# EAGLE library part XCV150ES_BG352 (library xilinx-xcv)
xcv150es_bg352 edit this description Auto generated by make-symbol-device-package-bsdl.ulp Rev. 26 Source: xcv150es_bg352.bsd
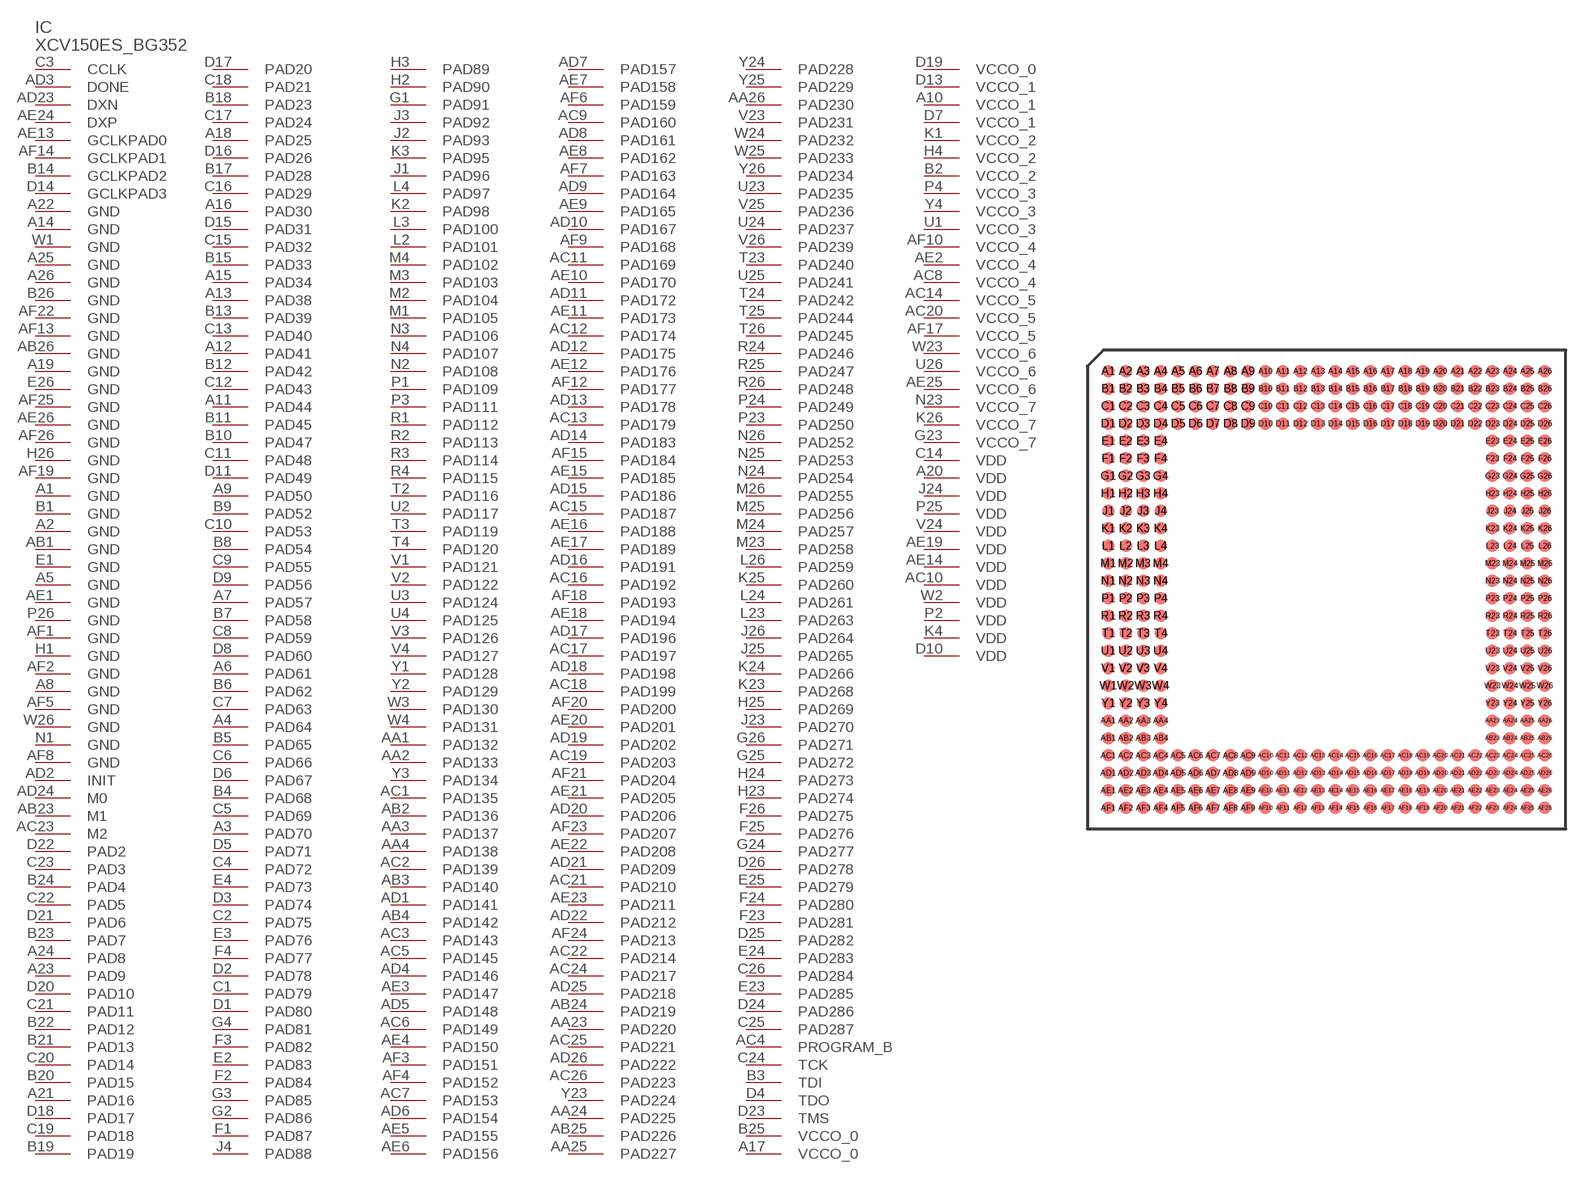
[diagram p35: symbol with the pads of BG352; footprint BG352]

Designator prefix IC

## XCV150ES_BG352 (OC_FARNELL: unknown; OC_NEWARK: unknown)  [BG352]
A1  GND  pwr
A2  GND  pwr
A3  PAD70
A4  PAD64
A5  GND  pwr
A6  PAD61
A7  PAD57
A8  GND  pwr
A9  PAD50
A10  VCCO_1  pwr
A11  PAD44
A12  PAD41
A13  PAD38
A14  GND  pwr
A15  PAD34
A16  PAD30
A17  VCCO_0  pwr
A18  PAD25
A19  GND  pwr
A20  VDD  pwr
A21  PAD16
A22  GND  pwr
A23  PAD9
A24  PAD8
A25  GND  pwr
A26  GND  pwr
AA1  PAD132
AA2  PAD133
AA3  PAD137
AA4  PAD138
AA23  PAD220
AA24  PAD225
AA25  PAD227
AA26  PAD230
AB1  GND  pwr
AB2  PAD136
AB3  PAD140
AB4  PAD142
AB23  M1  in
AB24  PAD219
AB25  PAD226
AB26  GND  pwr
AC1  PAD135
AC2  PAD139
AC3  PAD143
AC4  PROGRAM_B  in
AC5  PAD145
AC6  PAD149
AC7  PAD153
AC8  VCCO_4  pwr
AC9  PAD160
AC10  VDD  pwr
AC11  PAD169
AC12  PAD174
AC13  PAD179
AC14  VCCO_5  pwr
AC15  PAD187
AC16  PAD192
AC17  PAD197
AC18  PAD199
AC19  PAD203
AC20  VCCO_5  pwr
AC21  PAD210
AC22  PAD214
AC23  M2  in
AC24  PAD217
AC25  PAD221
AC26  PAD223
AD1  PAD141
AD2  INIT
AD3  DONE
AD4  PAD146
AD5  PAD148
AD6  PAD154
AD7  PAD157
AD8  PAD161
AD9  PAD164
AD10  PAD167
AD11  PAD172
AD12  PAD175
AD13  PAD178
AD14  PAD183
AD15  PAD186
AD16  PAD191
AD17  PAD196
AD18  PAD198
AD19  PAD202
AD20  PAD206
AD21  PAD209
AD22  PAD212
AD23  DXN  pas
AD24  M0  in
AD25  PAD218
AD26  PAD222
AE1  GND  pwr
AE2  VCCO_4  pwr
AE3  PAD147
AE4  PAD150
AE5  PAD155
AE6  PAD156
AE7  PAD158
AE8  PAD162
AE9  PAD165
AE10  PAD170
AE11  PAD173
AE12  PAD176
AE13  GCLKPAD0  in
AE14  VDD  pwr
AE15  PAD185
AE16  PAD188
AE17  PAD189
AE18  PAD194
AE19  VDD  pwr
AE20  PAD201
AE21  PAD205
AE22  PAD208
AE23  PAD211
AE24  DXP  pas
AE25  VCCO_6  pwr
AE26  GND  pwr
AF1  GND  pwr
AF2  GND  pwr
AF3  PAD151
AF4  PAD152
AF5  GND  pwr
AF6  PAD159
AF7  PAD163
AF8  GND  pwr
AF9  PAD168
AF10  VCCO_4  pwr
AF12  PAD177
AF13  GND  pwr
AF14  GCLKPAD1  in
AF15  PAD184
AF17  VCCO_5  pwr
AF18  PAD193
AF19  GND  pwr
AF20  PAD200
AF21  PAD204
AF22  GND  pwr
AF23  PAD207
AF24  PAD213
AF25  GND  pwr
AF26  GND  pwr
B1  GND  pwr
B2  VCCO_2  pwr
B3  TDI  in
B4  PAD68
B5  PAD65
B6  PAD62
B7  PAD58
B8  PAD54
B9  PAD52
B10  PAD47
B11  PAD45
B12  PAD42
B13  PAD39
B14  GCLKPAD2  in
B15  PAD33
B17  PAD28
B18  PAD23
B19  PAD19
B20  PAD15
B21  PAD13
B22  PAD12
B23  PAD7
B24  PAD4
B25  VCCO_0  pwr
B26  GND  pwr
C1  PAD79
C2  PAD75
C3  CCLK
C4  PAD72
C5  PAD69
C6  PAD66
C7  PAD63
C8  PAD59
C9  PAD55
C10  PAD53
C11  PAD48
C12  PAD43
C13  PAD40
C14  VDD  pwr
C15  PAD32
C16  PAD29
C17  PAD24
C18  PAD21
C19  PAD18
C20  PAD14
C21  PAD11
C22  PAD5
C23  PAD3
C24  TCK  in
C25  PAD287
C26  PAD284
D1  PAD80
D2  PAD78
D3  PAD74
D4  TDO  out
D5  PAD71
D6  PAD67
D7  VCCO_1  pwr
D8  PAD60
D9  PAD56
D10  VDD  pwr
D11  PAD49
D13  VCCO_1  pwr
D14  GCLKPAD3  in
D15  PAD31
D16  PAD26
D17  PAD20
D18  PAD17
D19  VCCO_0  pwr
D20  PAD10
D21  PAD6
D22  PAD2
D23  TMS  in
D24  PAD286
D25  PAD282
D26  PAD278
E1  GND  pwr
E2  PAD83
E3  PAD76
E4  PAD73
E23  PAD285
E24  PAD283
E25  PAD279
E26  GND  pwr
F1  PAD87
F2  PAD84
F3  PAD82
F4  PAD77
F23  PAD281
F24  PAD280
F25  PAD276
F26  PAD275
G1  PAD91
G2  PAD86
G3  PAD85
G4  PAD81
G23  VCCO_7  pwr
G24  PAD277
G25  PAD272
G26  PAD271
H1  GND  pwr
H2  PAD90
H3  PAD89
H4  VCCO_2  pwr
H23  PAD274
H24  PAD273
H25  PAD269
H26  GND  pwr
J1  PAD96
J2  PAD93
J3  PAD92
J4  PAD88
J23  PAD270
J24  VDD  pwr
J25  PAD265
J26  PAD264
K1  VCCO_2  pwr
K2  PAD98
K3  PAD95
K4  VDD  pwr
K23  PAD268
K24  PAD266
K25  PAD260
K26  VCCO_7  pwr
L2  PAD101
L3  PAD100
L4  PAD97
L23  PAD263
L24  PAD261
L26  PAD259
M1  PAD105
M2  PAD104
M3  PAD103
M4  PAD102
M23  PAD258
M24  PAD257
M25  PAD256
M26  PAD255
N1  GND  pwr
N2  PAD108
N3  PAD106
N4  PAD107
N23  VCCO_7  pwr
N24  PAD254
N25  PAD253
N26  PAD252
P1  PAD109
P2  VDD  pwr
P3  PAD111
P4  VCCO_3  pwr
P23  PAD250
P24  PAD249
P25  VDD  pwr
P26  GND  pwr
R1  PAD112
R2  PAD113
R3  PAD114
R4  PAD115
R24  PAD246
R25  PAD247
R26  PAD248
T2  PAD116
T3  PAD119
T4  PAD120
T23  PAD240
T24  PAD242
T25  PAD244
T26  PAD245
U1  VCCO_3  pwr
U2  PAD117
U3  PAD124
U4  PAD125
U23  PAD235
U24  PAD237
U25  PAD241
U26  VCCO_6  pwr
V1  PAD121
V2  PAD122
V3  PAD126
V4  PAD127
V23  PAD231
V24  VDD  pwr
V25  PAD236
V26  PAD239
W1  GND  pwr
W2  VDD  pwr
W3  PAD130
W4  PAD131
W23  VCCO_6  pwr
W24  PAD232
W25  PAD233
W26  GND  pwr
Y1  PAD128
Y2  PAD129
Y3  PAD134
Y4  VCCO_3  pwr
Y23  PAD224
Y24  PAD228
Y25  PAD229
Y26  PAD234

## Footprint BG352 (pad centres in mm)
xcv100e_bg352 edit this description Auto generated by make-symbol-device-package-bsdl.ulp Rev. 26 Source: xcv100e_bg352.bsd
smd 0.9 x 0.9: A1 -15.875,15.875; A2 -14.605,15.875; A3 -13.335,15.875; A4 -12.065,15.875; A5 -10.795,15.875; A6 -9.525,15.875; A7 -8.255,15.875; A8 -6.985,15.875; A9 -5.715,15.875; A10 -4.445,15.875; A11 -3.175,15.875; A12 -1.905,15.875; A13 -0.635,15.875; A14 0.635,15.875; A15 1.905,15.875; A16 3.175,15.875; A17 4.445,15.875; A18 5.715,15.875; A19 6.985,15.875; A20 8.255,15.875; A21 9.525,15.875; A22 10.795,15.875; A23 12.065,15.875; A24 13.335,15.875; A25 14.605,15.875; A26 15.875,15.875; AA1 -15.875,-9.525; AA2 -14.605,-9.525; AA3 -13.335,-9.525; AA4 -12.065,-9.525; AA23 12.065,-9.525; AA24 13.335,-9.525; AA25 14.605,-9.525; AA26 15.875,-9.525; AB1 -15.875,-10.795; AB2 -14.605,-10.795; AB3 -13.335,-10.795; AB4 -12.065,-10.795; AB23 12.065,-10.795; AB24 13.335,-10.795; AB25 14.605,-10.795; AB26 15.875,-10.795; AC1 -15.875,-12.065; AC2 -14.605,-12.065; AC3 -13.335,-12.065; AC4 -12.065,-12.065; AC5 -10.795,-12.065; AC6 -9.525,-12.065; AC7 -8.255,-12.065; AC8 -6.985,-12.065; AC9 -5.715,-12.065; AC10 -4.445,-12.065; AC11 -3.175,-12.065; AC12 -1.905,-12.065; AC13 -0.635,-12.065; AC14 0.635,-12.065; AC15 1.905,-12.065; AC16 3.175,-12.065; AC17 4.445,-12.065; AC18 5.715,-12.065; AC19 6.985,-12.065; AC20 8.255,-12.065; AC21 9.525,-12.065; AC22 10.795,-12.065; AC23 12.065,-12.065; AC24 13.335,-12.065; AC25 14.605,-12.065; AC26 15.875,-12.065; AD1 -15.875,-13.335; AD2 -14.605,-13.335; AD3 -13.335,-13.335; AD4 -12.065,-13.335; AD5 -10.795,-13.335; AD6 -9.525,-13.335; AD7 -8.255,-13.335; AD8 -6.985,-13.335; AD9 -5.715,-13.335; AD10 -4.445,-13.335; AD11 -3.175,-13.335; AD12 -1.905,-13.335; AD13 -0.635,-13.335; AD14 0.635,-13.335; AD15 1.905,-13.335; AD16 3.175,-13.335; AD17 4.445,-13.335; AD18 5.715,-13.335; AD19 6.985,-13.335; AD20 8.255,-13.335; AD21 9.525,-13.335; AD22 10.795,-13.335; AD23 12.065,-13.335; AD24 13.335,-13.335; AD25 14.605,-13.335; AD26 15.875,-13.335; AE1 -15.875,-14.605; AE2 -14.605,-14.605; AE3 -13.335,-14.605; AE4 -12.065,-14.605; AE5 -10.795,-14.605; AE6 -9.525,-14.605; AE7 -8.255,-14.605; AE8 -6.985,-14.605; AE9 -5.715,-14.605; AE10 -4.445,-14.605; AE11 -3.175,-14.605; AE12 -1.905,-14.605; AE13 -0.635,-14.605; AE14 0.635,-14.605; AE15 1.905,-14.605; AE16 3.175,-14.605; AE17 4.445,-14.605; AE18 5.715,-14.605; AE19 6.985,-14.605; AE20 8.255,-14.605; AE21 9.525,-14.605; AE22 10.795,-14.605; AE23 12.065,-14.605; AE24 13.335,-14.605; AE25 14.605,-14.605; AE26 15.875,-14.605; AF1 -15.875,-15.875; AF2 -14.605,-15.875; AF3 -13.335,-15.875; AF4 -12.065,-15.875; AF5 -10.795,-15.875; AF6 -9.525,-15.875; AF7 -8.255,-15.875; AF8 -6.985,-15.875; AF9 -5.715,-15.875; AF10 -4.445,-15.875; AF11 -3.175,-15.875; AF12 -1.905,-15.875; AF13 -0.635,-15.875; AF14 0.635,-15.875; AF15 1.905,-15.875; AF16 3.175,-15.875; AF17 4.445,-15.875; AF18 5.715,-15.875; AF19 6.985,-15.875; AF20 8.255,-15.875; AF21 9.525,-15.875; AF22 10.795,-15.875; AF23 12.065,-15.875; AF24 13.335,-15.875; AF25 14.605,-15.875; AF26 15.875,-15.875; B1 -15.875,14.605; B2 -14.605,14.605; B3 -13.335,14.605; B4 -12.065,14.605; B5 -10.795,14.605; B6 -9.525,14.605; B7 -8.255,14.605; B8 -6.985,14.605; B9 -5.715,14.605; B10 -4.445,14.605; B11 -3.175,14.605; B12 -1.905,14.605; B13 -0.635,14.605; B14 0.635,14.605; B15 1.905,14.605; B16 3.175,14.605; B17 4.445,14.605; B18 5.715,14.605; B19 6.985,14.605; B20 8.255,14.605; B21 9.525,14.605; B22 10.795,14.605; B23 12.065,14.605; B24 13.335,14.605; B25 14.605,14.605; B26 15.875,14.605; C1 -15.875,13.335; C2 -14.605,13.335; C3 -13.335,13.335; C4 -12.065,13.335; C5 -10.795,13.335; C6 -9.525,13.335; C7 -8.255,13.335; C8 -6.985,13.335; C9 -5.715,13.335; C10 -4.445,13.335; C11 -3.175,13.335; C12 -1.905,13.335; C13 -0.635,13.335; C14 0.635,13.335; C15 1.905,13.335; C16 3.175,13.335; C17 4.445,13.335; C18 5.715,13.335; C19 6.985,13.335; C20 8.255,13.335; C21 9.525,13.335; C22 10.795,13.335; C23 12.065,13.335; C24 13.335,13.335; C25 14.605,13.335; C26 15.875,13.335; D1 -15.875,12.065; D2 -14.605,12.065; D3 -13.335,12.065; D4 -12.065,12.065; D5 -10.795,12.065; D6 -9.525,12.065; D7 -8.255,12.065; D8 -6.985,12.065; D9 -5.715,12.065; D10 -4.445,12.065; D11 -3.175,12.065; D12 -1.905,12.065; D13 -0.635,12.065; D14 0.635,12.065; D15 1.905,12.065; D16 3.175,12.065; D17 4.445,12.065; D18 5.715,12.065; D19 6.985,12.065; D20 8.255,12.065; D21 9.525,12.065; D22 10.795,12.065; D23 12.065,12.065; D24 13.335,12.065; D25 14.605,12.065; D26 15.875,12.065; E1 -15.875,10.795; E2 -14.605,10.795; E3 -13.335,10.795; E4 -12.065,10.795; E23 12.065,10.795; E24 13.335,10.795; E25 14.605,10.795; E26 15.875,10.795; F1 -15.875,9.525; F2 -14.605,9.525; F3 -13.335,9.525; F4 -12.065,9.525; F23 12.065,9.525; F24 13.335,9.525; F25 14.605,9.525; F26 15.875,9.525; G1 -15.875,8.255; G2 -14.605,8.255; G3 -13.335,8.255; G4 -12.065,8.255; G23 12.065,8.255; G24 13.335,8.255; G25 14.605,8.255; G26 15.875,8.255; H1 -15.875,6.985; H2 -14.605,6.985; H3 -13.335,6.985; H4 -12.065,6.985; H23 12.065,6.985; H24 13.335,6.985; H25 14.605,6.985; H26 15.875,6.985; J1 -15.875,5.715; J2 -14.605,5.715; J3 -13.335,5.715; J4 -12.065,5.715; J23 12.065,5.715; J24 13.335,5.715; J25 14.605,5.715; J26 15.875,5.715; K1 -15.875,4.445; K2 -14.605,4.445; K3 -13.335,4.445; K4 -12.065,4.445; K23 12.065,4.445; K24 13.335,4.445; K25 14.605,4.445; K26 15.875,4.445; L1 -15.875,3.175; L2 -14.605,3.175; L3 -13.335,3.175; L4 -12.065,3.175; L23 12.065,3.175; L24 13.335,3.175; L25 14.605,3.175; L26 15.875,3.175; M1 -15.875,1.905; M2 -14.605,1.905; M3 -13.335,1.905; M4 -12.065,1.905; M23 12.065,1.905; M24 13.335,1.905; M25 14.605,1.905; M26 15.875,1.905; N1 -15.875,0.635; N2 -14.605,0.635; N3 -13.335,0.635; N4 -12.065,0.635; N23 12.065,0.635; N24 13.335,0.635; N25 14.605,0.635; N26 15.875,0.635; P1 -15.875,-0.635; P2 -14.605,-0.635; P3 -13.335,-0.635; P4 -12.065,-0.635; P23 12.065,-0.635; P24 13.335,-0.635; P25 14.605,-0.635; P26 15.875,-0.635; R1 -15.875,-1.905; R2 -14.605,-1.905; R3 -13.335,-1.905; R4 -12.065,-1.905; R23 12.065,-1.905; R24 13.335,-1.905; R25 14.605,-1.905; R26 15.875,-1.905; T1 -15.875,-3.175; T2 -14.605,-3.175; T3 -13.335,-3.175; T4 -12.065,-3.175; T23 12.065,-3.175; T24 13.335,-3.175; T25 14.605,-3.175; T26 15.875,-3.175; U1 -15.875,-4.445; U2 -14.605,-4.445; U3 -13.335,-4.445; U4 -12.065,-4.445; U23 12.065,-4.445; U24 13.335,-4.445; U25 14.605,-4.445; U26 15.875,-4.445; V1 -15.875,-5.715; V2 -14.605,-5.715; V3 -13.335,-5.715; V4 -12.065,-5.715; V23 12.065,-5.715; V24 13.335,-5.715; V25 14.605,-5.715; V26 15.875,-5.715; W1 -15.875,-6.985; W2 -14.605,-6.985; W3 -13.335,-6.985; W4 -12.065,-6.985; W23 12.065,-6.985; W24 13.335,-6.985; W25 14.605,-6.985; W26 15.875,-6.985; Y1 -15.875,-8.255; Y2 -14.605,-8.255; Y3 -13.335,-8.255; Y4 -12.065,-8.255; Y23 12.065,-8.255; Y24 13.335,-8.255; Y25 14.605,-8.255; Y26 15.875,-8.255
